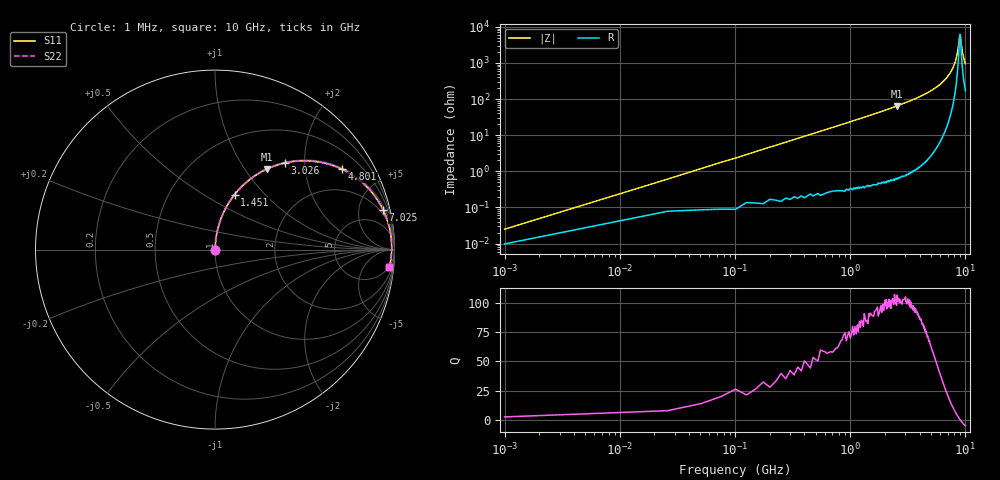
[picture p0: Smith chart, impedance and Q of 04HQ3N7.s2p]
! Coilcraft 0403HQ-3N7 Chip Inductor
! 13 February 2004
# MHZ S MA R 50
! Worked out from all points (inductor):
!   401 points, 1 MHz to 10 GHz, reference 50 ohm
!   read as one part in series: L = 3.72 nH near 50.99 MHz
!   highest Q = 103 at 2.526 GHz (marker M1), where L = 4.02 nH
!   self-resonance near 8.975 GHz
!   S11 on the Smith chart (normalised r, x): 1 MHz: 1.00, +0.00; 1.451 GHz: 1.01, +0.69; 3.026 GHz: 1.01, +1.59; 4.801 GHz: 1.04, +3.13; 7.025 GHz: 1.39, +8.42; 10 GHz: 4, -19
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1  0.0003036 49.9  1 -0.0  1 -0.0  0.0003036 49.9
75.992  0.018 86.0  0.999 -1.0  0.999 -1.0  0.018 86.0
150.985  0.035 85.9  0.998 -2.0  0.998 -2.0  0.035 85.9
250.975  0.058 85.1  0.997 -3.3  0.997 -3.3  0.058 85.1
450.955  0.104 82.8  0.992 -6.0  0.992 -6.0  0.104 82.8
700.93  0.161 79.8  0.984 -9.3  0.984 -9.3  0.161 79.8
1450.855  0.326 70.3  0.942 -19.0  0.942 -19.0  0.326 70.3
1675.832  0.373 67.5  0.924 -21.9  0.924 -21.9  0.373 67.5
2525.747  0.535 57.1  0.839 -32.4  0.839 -32.4  0.535 57.1
3025.697  0.619 51.2  0.78 -38.2  0.78 -38.2  0.619 51.2
3350.665  0.668 47.5  0.738 -41.9  0.738 -41.9  0.668 47.5
4800.52  0.837 32.4  0.535 -56.8  0.535 -56.8  0.837 32.4
5000.5  0.854 30.4  0.507 -58.7  0.507 -58.7  0.854 30.4
6675.333  0.951 15.9  0.274 -71.9  0.274 -71.9  0.951 15.9
7025.298  0.963 13.2  0.229 -74.0  0.229 -74.0  0.963 13.2
7800.22  0.979 7.6  0.133 -76.9  0.133 -76.9  0.979 7.6
8350.165  0.984 3.9  0.07 -74.5  0.07 -74.5  0.984 3.9
8625.138  0.985 2.2  0.041 -66.6  0.041 -66.6  0.985 2.2
8875.113  0.985 0.6  0.019 -34.7  0.019 -34.7  0.985 0.6
8975.103  0.984 0.0  0.016 -1.1  0.016 -1.1  0.984 0.0
9475.053  0.982 -2.9  0.053 68.6  0.053 68.6  0.982 -2.9
10000  0.976 -5.8  0.103 73.9  0.103 73.9  0.976 -5.8
